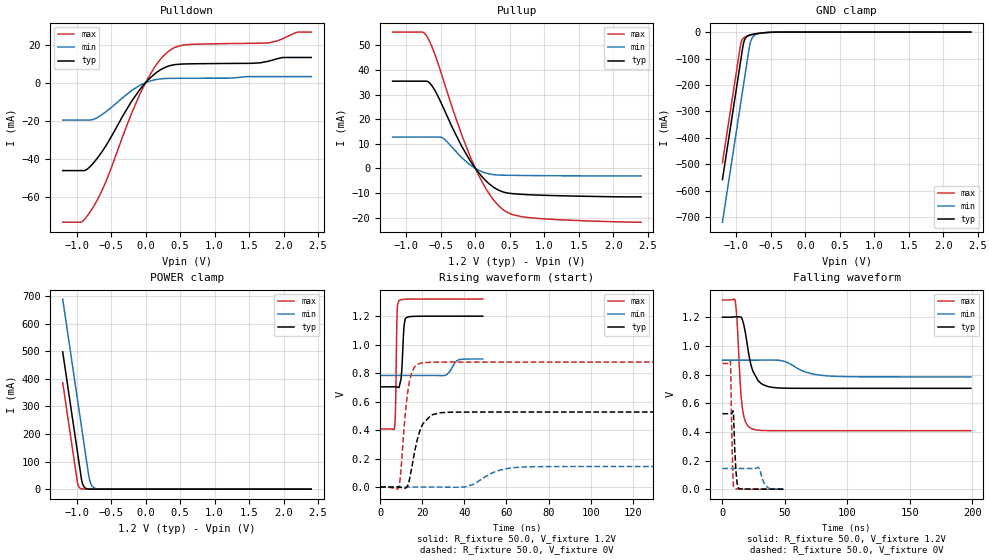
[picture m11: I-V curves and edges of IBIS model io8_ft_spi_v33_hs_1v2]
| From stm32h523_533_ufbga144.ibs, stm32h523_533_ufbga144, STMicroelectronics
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[Model]   io8_ft_spi_v33_hs_1v2
Model_type I/O
Polarity   Non-Inverting
Enable   Active-Low
| CAP_THRESHOLD on pad IOFT is "UDTCAPC" :
| Rising=20.0% of vddiom   Falling=80.0% of vddiom
| C_comp min and max val. don't necessarily correlate with the min and max pvt
| but are the smallest and greatest pad capacitance found.
| var   typ   min   max
C_comp   3.39520pF  3.36985pF  3.42670pF
|C_comp_pullup   2.08425pF  1.99555pF  1.90045pF
|C_comp_pulldown   1.31095pF  1.37430pF  1.52625pF
Vinl = 270.0mV
Vinh = 924.0mV
Vmeas = 600.0mV   | Reference voltage for timing measurements
Cref  = 50.0pF   | Timing specification test load capacitance value
Rref  = 100.0MOhm   | Timing specification test load resistance value
Vref  = 600.0mV   | Timing specification test load voltage
[Model Spec]
| TIME_THRESHOLD on pin ZIV33M is "CMOS" :
| Rising=40.0% of vddiom   Falling=60.0% of vddiom
Vinl 437.80000mV 335.80000mV 479.80000mV
Vinh 728.20000mV 529.20000mV 807.20000mV
| variable   typ   min   max
[Temperature Range] 25.0 125.0 -40.0
| variable   typ   min   max
[Voltage Range] 1.2V 900.0mV 1.32V
| variable   typ   min   max
[POWER Clamp Reference] 1.2V 900.0mV 1.32V
| variable   typ   min   max
[GND Clamp Reference] 0V 0V 0V
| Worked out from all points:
|   slope of the pulldown table from 0 to 0.18 V, typ, clamps not added: 30.6 ohm
|   slope of the pullup table from 0 to 0.18 V, typ, clamps not added: 31.2 ohm
|   GND clamp passes 1 mA (typ) near -0.52 V on its own axis
|   POWER clamp passes 1 mA (typ) near -0.84 V on its own axis
|   rising waveform, R_fixture 50.0, V_fixture 1.2V: 20-80 % time 1.03ns typ, 2.95ns min, 549ps max; typ from 0.704 V to 1.2 V
|   falling waveform, R_fixture 50.0, V_fixture 1.2V: 20-80 % time 7.52ns typ, 17.2ns min, 3.69ns max; typ from 1.2 V to 0.704 V
|   rising waveform, R_fixture 50.0, V_fixture 0V: 20-80 % time 4.98ns typ, 10.7ns min, 3.3ns max; typ from 0 V to 0.527 V
|   falling waveform, R_fixture 50.0, V_fixture 0V: 20-80 % time 1.75ns typ, 3.87ns min, 1.25ns max; typ from 0.527 V to 0 V
[POWER Clamp]
-1.2V     497.8mA    689.2mA    386.5mA
-990mV    140.8mA    332.2mA    29.53mA
-980mV    123.8mA    315.2mA    17.95mA
-960mV    89.81mA    281.2mA    6.634mA
-930mV    38.81mA    230.2mA    1.49mA
-900mV    12.07mA    179.2mA    334.8uA
-870mV    3.756mA    128.2mA    75.22uA
-820mV    536.4uA    44.98mA    6.246uA
-790mV    166.9uA    18.76mA    1.403uA
-750mV    35.18uA    5.846mA    191.8nA
-590mV    70.09nA    55uA       165.5pA
2.4V      0A         0A         0A
[GND Clamp]
-1.2V     -558.2mA   -719mA     -494.1mA
-940mV    -116.2mA   -277mA     -52.06mA
-930mV    -99.19mA   -260mA     -39.94mA
-900mV    -49.1mA    -209mA     -23.76mA
-880mV    -30.14mA   -175mA     -19.6mA
-850mV    -17.82mA   -124mA     -16.09mA
-810mV    -11.73mA   -56.78mA   -12.91mA
-780mV    -9.444mA   -28.21mA   -10.92mA
-740mV    -7.291mA   -13.16mA   -8.574mA
-640mV    -3.573mA   -4.171mA   -3.954mA
-380mV    -61.75uA   -230.3uA   -20.32uA
2.4V      3.863nA    718.4nA    150.6pA
| variable   typ   min   max
[Pullup Reference] 1.2V 900.0mV 1.32V
| variable   typ   min   max
[Pulldown Reference] 0V 0V 0V
[Pullup]
-1.2V     35.45mA    12.72mA    55.38mA
-770mV    35.45mA    12.72mA    55.38mA
-700mV    35.4mA     12.72mA    53.49mA
-610mV    32.76mA    12.72mA    48.02mA
-470mV    25.02mA    12.31mA    36.49mA
-200mV    9.076mA    4.406mA    13.76mA
0V        5.98pA     656pA      2.91pA
200mV     -6.256mA   -2.236mA   -10.31mA
400mV     -9.528mA   -2.741mA   -16.71mA
540mV     -10.25mA   -2.811mA   -18.8mA
790mV     -10.7mA    -2.892mA   -20.02mA
2.4V      -11.55mA   -3.057mA   -21.84mA
[Pulldown]
-1.2V     -46.17mA   -19.62mA   -73.27mA
-930mV    -46.17mA   -19.62mA   -73.18mA
-770mV    -42.8mA    -19.41mA   -66.04mA
-570mV    -32.88mA   -15.18mA   -51.58mA
-200mV    -9.658mA   -4.084mA   -15.89mA
-80mV     -3.488mA   -1.363mA   -5.887mA
120mV     4.232mA    1.387mA    7.501mA
340mV     8.782mA    2.251mA    16.66mA
540mV     9.805mA    2.305mA    19.74mA
1.79V     11.33mA    3.206mA    20.93mA
2.2V      13.23mA    3.206mA    26.48mA
2.4V      13.23mA    3.206mA    26.56mA
[Ramp]
dV/dt_r 315.96819mV/4.93963ns 86.45003mV/10.53483ns 526.3454mV/3.29267ns
dV/dt_f 297.8052mV/7.1315ns 69.92235mV/16.99961ns 547.1393mV/3.65761ns
R_load = 50.0
| Removed startup time: 0s 0s 0s  .
| Removed end time: 48.75ns.
[Rising Waveform]
R_fixture   = 50.0
V_fixture   = 1.2V
V_fixture_min = 900.0mV
V_fixture_max = 1.32V
0s        703.7mV    783.5mV    408.1mV
6.8ns     703.8mV    783.5mV    414.3mV
7.3ns     703.8mV    783.5mV    553.7mV
8.05ns    702mV      783.5mV    1.219V
8.95ns    698.4mV    783.5mV    1.31V
9.95ns    759.9mV    783.5mV    1.315V
11.2ns    1.1V       783.5mV    1.318V
11.95ns   1.183V     783.5mV    1.319V
30.85ns   1.2V       784mV      1.32V
48.75ns   1.2V       899.2mV    1.32V
| Removed startup time: 0s 0s 0s  .
| Removed end time: 198.75ns.
[Falling Waveform]
R_fixture   = 50.0
V_fixture   = 1.2V
V_fixture_min = 900.0mV
V_fixture_max = 1.32V
0s        1.2V       900mV      1.32V
10.15ns   1.203V     900mV      1.32V
11.8ns    1.203V     900mV      1.158V
14.4ns    1.201V     900mV      715mV
16.25ns   1.173V     900mV      546.8mV
23.45ns   847.9mV    900mV      421.8mV
30.85ns   738.2mV    901.2mV    409.9mV
40.55ns   709.6mV    900.8mV    408.2mV
81.15ns   703.7mV    792.6mV    408.1mV
198.8ns   703.7mV    783.5mV    408.1mV
| Removed startup time: 0s 0s 0s  .
| Removed end time: 198.7ns.
[Rising Waveform]
R_fixture   = 50.0
V_fixture   = 0V
V_fixture_min = 0V
V_fixture_max = 0V
0s        202.1nV    701.3nV    137.6nV
8.9ns     -276.8uV   707.4nV    2.732mV
12.1ns    -7.081mV   697.8nV    535.8mV
13.6ns    32.55mV    685.4nV    715mV
16.2ns    233.5mV    986.3nV    839.9mV
18.8ns    391.4mV    950.7nV    867.8mV
24.3ns    505.5mV    -341.7nV   876.5mV
32.5ns    525.1mV    -1.359mV   877.1mV
64.9ns    526.5mV    137.7mV    877.2mV
198.7ns   526.6mV    144.1mV    877.2mV
| Removed startup time: 0s 0s 0s  .
| Removed end time: 48.75ns.
[Falling Waveform]
R_fixture   = 50.0
V_fixture   = 0V
V_fixture_min = 0V
V_fixture_max = 0V
0s        526.7mV    144.2mV    877.3mV
6.4ns     526.5mV    144.2mV    890.4mV
7.95ns    534.8mV    144.2mV    222mV
8.7ns     539.6mV    144.2mV    40.15mV
9.35ns    406.9mV    144.2mV    9.639mV
10.95ns   113.3mV    144.2mV    2.891mV
12.95ns   4.926mV    144.2mV    1.1mV
28.9ns    116.9uV    151.5mV    9.46uV
35.85ns   32.02uV    14.7mV     1.346uV
48.75ns   2.433uV    567.4uV    55.95nV
